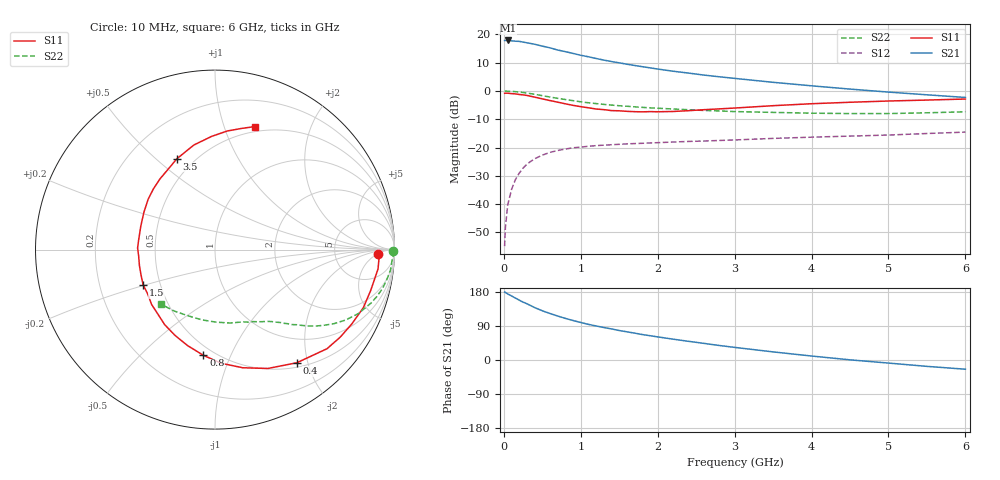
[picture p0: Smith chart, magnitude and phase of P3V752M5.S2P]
! SIEMENS Small Signal Semiconductors
! BFP181
! Si NPN RF Bipolar Junction Transistor in SOT143
! VCE = 0.75 V  IC = 2.5 mA
! Common Emitter S-Parameters:  March  1996
# GHz  S  MA  R  50
!  f  S11  S21  S12  S22
! GHz  MAG  ANG  MAG  ANG  MAG  ANG  MAG  ANG
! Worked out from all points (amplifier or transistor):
!   36 points, 10 MHz to 6 GHz, reference 50 ohm
!   highest |S21| = 17.9 dB at 50 MHz (marker M1)
!   |S21| within 3 dB of that: start of sweep to 650 MHz
!   unconditionally stable (mu >= 1): 1.972 GHz to end of sweep
!   at 250 MHz: K = 0.16, MSG = 22.3 dB, |S12| = -27.3 dB
!   at 1.4 GHz: K = 0.78, MSG = 14.7 dB, |S12| = -19.0 dB
!   at 6 GHz: K = 1.22, MAG = 3.3 dB, |S12| = -14.6 dB
!   S11 on the Smith chart (normalised r, x): 10 MHz: 19, -6; 400 MHz: 0.57, -1.82; 800 MHz: 0.44, -0.80; 1.5 GHz: 0.40, -0.20; 3.5 GHz: 0.40, +0.59; 6 GHz: 0.45, +1.27
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0.01  0.9087 -1.6  7.81 179.2  0.0018 86.8  0.993 -0.6
0.02  0.9153 -2.9  7.797 178.3  0.0038 86.5  0.9955 -1.3
0.05  0.9146 -6.8  7.818 174.5  0.0096 88.1  0.9887 -3.4
0.1  0.897 -14.6  7.695 169.0  0.0181 81.1  0.984 -6.8
0.2  0.8673 -28.6  7.533 158.0  0.0352 73.4  0.9572 -13.2
0.25  0.8512 -35.0  7.315 152.8  0.0432 69.3  0.9379 -16.3
0.4  0.7782 -54.1  6.705 138.4  0.0632 59.1  0.874 -24.1
0.5  0.7249 -66.0  6.209 129.9  0.0733 53.3  0.8258 -28.4
0.6  0.6762 -76.8  5.785 122.7  0.0821 48.6  0.781 -31.9
0.7  0.6341 -86.9  5.295 116.0  0.0885 44.6  0.7404 -34.7
0.8  0.5923 -96.3  4.957 109.8  0.0939 41.0  0.7059 -37.1
0.9  0.5563 -105.9  4.61 104.2  0.0989 37.9  0.6734 -39.2
1.1  0.5034 -123.9  4.022 94.0  0.1052 33.3  0.6184 -42.6
1.3  0.4672 -139.1  3.513 85.7  0.1101 29.6  0.579 -45.5
1.5  0.4459 -153.9  3.142 77.8  0.1139 27.0  0.5479 -47.9
1.8  0.4269 -175.1  2.687 67.2  0.1187 24.5  0.513 -51.5
2.2  0.4336 162.4  2.234 55.0  0.125 21.5  0.48 -56.8
2.8  0.4818 135.5  1.781 38.3  0.1331 18.7  0.4434 -65.7
3.5  0.5491 112.7  1.422 21.4  0.1449 15.7  0.4179 -78.2
4.5  0.6311 91.7  1.079 0.4  0.1591 11.1  0.3983 -100.5
5.5  0.6903 77.8  0.855 -16.8  0.1769 7.7  0.411 -123.7
6  0.7202 72.1  0.768 -24.3  0.1871 5.1  0.4284 -135.1
